(* Logix 5000 AddOnInstructionDefinition export AMCI_MAFR; software revision 20.05 *)

TYPE AMCI_Motion_Axis_Output_Data :
STRUCT
   Control_Word_0 : INT;
   Control_Word_1 : INT;
   Position_or_Distance : DINT;
   Programmed_Speed : DINT;
   Acceleration : INT;
   Deceleration : INT;
   Output_Word_8 : INT;
   Output_Word_9 : INT;
END_STRUCT
END_TYPE

TYPE AMCI_Motion_Axis_Input_Data :
STRUCT
   Moving_CW : BOOL;
   Moving_CCW : BOOL;
   In_Hold_State : BOOL;
   Stopped : BOOL;
   At_Home : BOOL;
   Accelerating : BOOL;
   Decelerating : BOOL;
   Move_Complete : BOOL;
   Status_Word_0_Bit_8 : BOOL;
   Status_Word_0_Bit_9 : BOOL;
   Position_Invalid : BOOL;
   Input_Error : BOOL;
   Command_Error : BOOL;
   Configuration_Error : BOOL;
   Module_OK : BOOL;
   Mode_Flag : BOOL;
   IN1_Active : BOOL;
   IN2_Active : BOOL;
   IN3_Active : BOOL;
   IN4_Active : BOOL;
   Status_Word_1_Bit_4 : BOOL;
   Status_Word_1_Bit_5 : BOOL;
   Connection_Was_Lost : BOOL;
   Driver_Fault : BOOL;
   Status_Word_1_Bit_8 : BOOL;
   Invalid_Jog_Change : BOOL;
   Status_Word_1_Bit_10 : BOOL;
   Heartbeat_Bit : BOOL;
   Status_Word_1_Bit_12 : BOOL;
   Status_Word_1_Bit_13 : BOOL;
   Stall_Detected : BOOL;
   Drive_Is_Enabled : BOOL;
   Motor_Position : DINT;
   Encoder_Position : DINT;
   Trapped_Encoder_Position : DINT;
   Input_Word_8 : INT;
   Input_Word_9 : INT;
END_STRUCT
END_TYPE

ADD_ON_INSTRUCTION AMCI_MAFR   (* revision 1.1, vendor AMCI, ExecuteEnableInFalse *)
// AMCI Reset Errors
// Revision note:
// V1.1 11/17/23 Reset output word 0 to 0 when the rung goes false.
// Help:
// MOTION AXIS FAULT RESET:   Resets Command, Input, and Stall Detect Errors.  It will also reset the Move Complete Status Bit.
// Note: This instruction will maintain the motion device’s current enabled state.  That is, if the device is enabled,
//            it will remain enabled.  If it is disabled, it will remain disabled.
// AXIS INPUT DATA:  Input data from AMCI motion device.   Uses the AMCI_Motion_Axis_Input_Data User Defined Data Type.
// AXIS OUTPUT DATA; Output data from the AOI to the AMCI motion device.   Uses the AMCI_Motion_Axis_Output_Data User Defined Data Type.
// EN (Enable) Set when rung is true, Reset when rung is false
// DN (Done) Set when command is sent to the motion device.  Reset when the rung is false.
// ER (Error) Set when a command or input error failed to clear.  Reset when the rung is false.
VAR_IN_OUT
   Axis_Input_Data : AMCI_Motion_Axis_Input_Data; {required}
        [0].6   // set when decelerating
   Axis_Output_Data : AMCI_Motion_Axis_Output_Data; {required}
END_VAR
VAR_OUTPUT
   EN : BOOL; {visible}   // set when rung with AOI is true
   DN : BOOL; {access Read Only, visible}   // set when reset error command sent to motion axis
   ER : BOOL; {access Read Only, visible}   // set when reset error command did not clear the error
END_VAR
VAR
   command_data_block : INT[10];
        [0]   // Command Bits MSW
        [1]   // Command Bits LSW
        [2]   // Upper Target Position
        [3]   // Lower Target Position
        [4]   // Upper Programmed Speed
        [5]   // Lower Programmed Speed
END_VAR

ROUTINE EnableInFalse   (* ladder *)
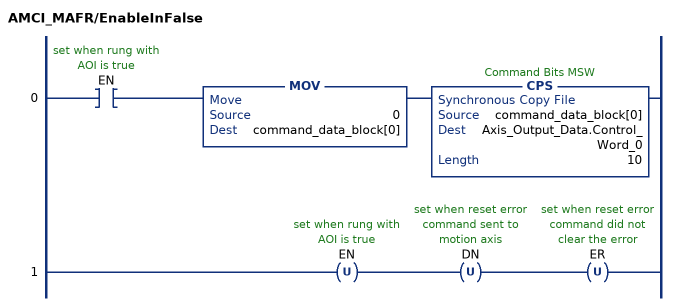
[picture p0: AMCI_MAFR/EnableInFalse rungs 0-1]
   0: XIC(EN)MOV(0,command_data_block[0])CPS(command_data_block[0],Axis_Output_Data.Control_Word_0,10);
   1: OTU(EN)OTU(DN)OTU(ER);
END_ROUTINE

ROUTINE Logic   (* ladder *)
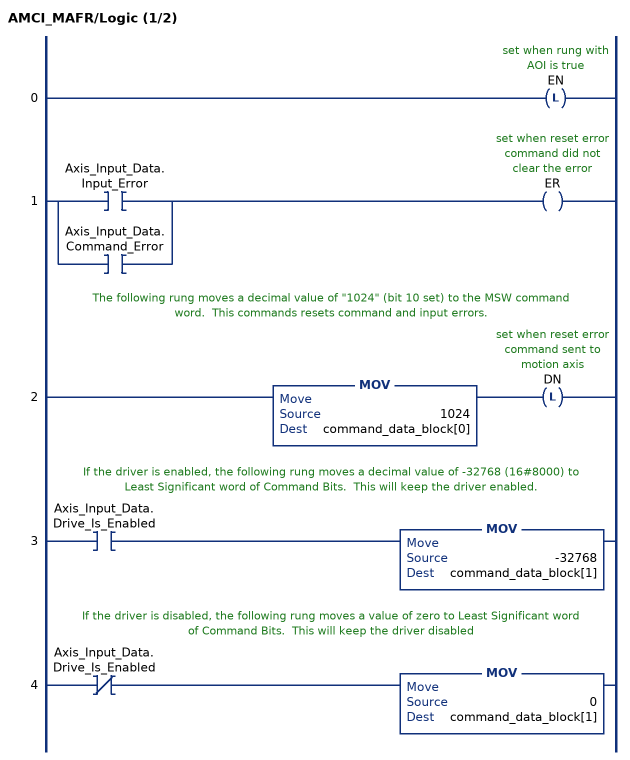
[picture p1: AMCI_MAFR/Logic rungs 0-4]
   0: OTL(EN);
   1: [XIC(Axis_Input_Data.Input_Error) ,XIC(Axis_Input_Data.Command_Error) ]OTE(ER);
   // The following rung moves a decimal value of "1024" (bit 10 set) to the MSW command word.  This commands resets command and input errors.
   2: MOV(1024,command_data_block[0])OTL(DN);
   // If the driver is enabled, the following rung moves a decimal value of -32768 (16#8000) to Least Significant word of Command Bits.  This will keep the driver enabled.
   3: XIC(Axis_Input_Data.Drive_Is_Enabled)MOV(-32768,command_data_block[1]);
   // If the driver is disabled, the following rung moves a value of zero to Least Significant word of Command Bits.  This will keep the driver disabled
   4: XIO(Axis_Input_Data.Drive_Is_Enabled)MOV(0,command_data_block[1]);
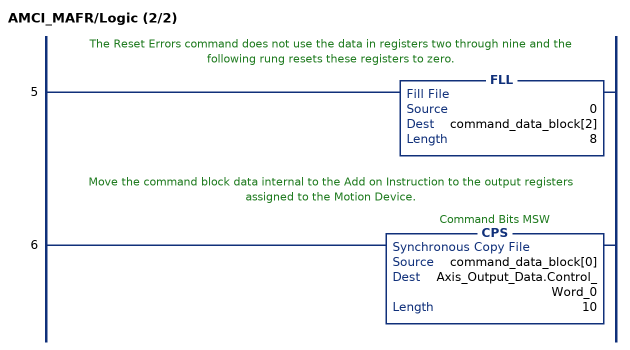
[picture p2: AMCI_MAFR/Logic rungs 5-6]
   // The Reset Errors command does not use the data in registers two through nine and the following rung resets these registers to zero.
   5: FLL(0,command_data_block[2],8);
   // Move the command block data internal to the Add on Instruction to the output registers assigned to the Motion Device.
   6: CPS(command_data_block[0],Axis_Output_Data.Control_Word_0,10);
END_ROUTINE
END_ADD_ON_INSTRUCTION
